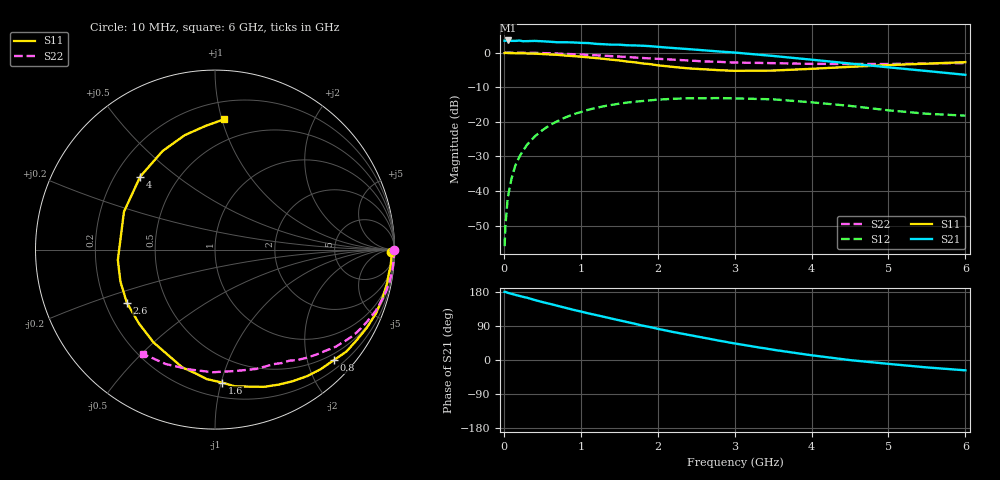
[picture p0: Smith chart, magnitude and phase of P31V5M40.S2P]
! SIEMENS Small Signal Semiconductors
! BFP181
! Si NPN RF Bipolar Junction Transistor in SOT143
! VCE = 1.5 V  IC = 0.4 mA
! Common Emitter S-Parameters:  March  1996
# GHz  S  MA  R  50
!  f  S11  S21  S12  S22
! GHz  MAG  ANG  MAG  ANG  MAG  ANG  MAG  ANG
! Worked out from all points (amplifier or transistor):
!   36 points, 10 MHz to 6 GHz, reference 50 ohm
!   highest |S21| = 3.5 dB at 50 MHz (marker M1)
!   |S21| within 3 dB of that: start of sweep to 2.69 GHz
!   unconditionally stable (mu >= 1): 3.807 GHz to end of sweep
!   at 250 MHz: K = 0.07, MSG = 15.8 dB, |S12| = -28.3 dB
!   at 1.4 GHz: K = 0.44, MSG = 8.7 dB, |S12| = -15.1 dB
!   at 6 GHz: K = 1.54, MAG = 1.6 dB, |S12| = -18.2 dB
!   S11 on the Smith chart (normalised r, x): 10 MHz: 76, -51; 800 MHz: 0.37, -2.50; 1.6 GHz: 0.31, -1.01; 2.6 GHz: 0.29, -0.26; 4 GHz: 0.30, +0.37; 6 GHz: 0.33, +1.01
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0.01  0.9821 -0.7  1.481 179.9  0.0016 87.2  0.9998 -0.2
0.02  0.9895 -1.2  1.482 179.7  0.0031 88.7  0.9928 -0.5
0.05  0.9844 -2.5  1.495 177.4  0.0079 90.7  0.9989 -1.4
0.1  0.9824 -5.5  1.475 174.7  0.0151 86.0  0.9975 -2.7
0.15  0.9773 -8.2  1.472 171.9  0.0235 84.6  0.9964 -4.0
0.2  0.9772 -10.8  1.49 169.2  0.031 81.9  0.9954 -5.4
0.3  0.9711 -16.3  1.461 164.5  0.0463 78.1  0.9931 -8.0
0.5  0.9514 -27.2  1.455 152.9  0.0755 70.4  0.9821 -13.3
0.8  0.9044 -42.9  1.408 137.8  0.1156 58.7  0.9582 -20.9
1.1  0.8514 -59.5  1.371 123.0  0.1495 47.7  0.9244 -28.2
1.3  0.8117 -70.4  1.319 114.0  0.1677 40.9  0.9012 -32.7
1.5  0.77 -81.7  1.3 104.8  0.1826 34.6  0.8744 -36.8
1.6  0.742 -86.9  1.274 100.3  0.1895 31.9  0.8646 -38.6
1.9  0.6806 -105.6  1.237 86.9  0.204 22.8  0.8225 -44.5
2.2  0.6203 -123.5  1.162 73.9  0.2149 14.9  0.7902 -49.7
2.6  0.5733 -149.0  1.078 58.7  0.2187 5.3  0.7448 -56.2
3  0.5444 -173.9  1 43.7  0.2179 -4.2  0.7172 -62.8
3.5  0.5494 157.4  0.893 27.1  0.2112 -13.6  0.7035 -70.9
4  0.5823 135.7  0.789 12.5  0.1911 -21.3  0.6859 -80.5
4.5  0.622 118.0  0.694 -0.3  0.1697 -27.1  0.6834 -91.1
5.5  0.6914 94.3  0.541 -19.6  0.1306 -26.3  0.6938 -113.2
6  0.7272 86.1  0.477 -27.3  0.1227 -21.4  0.7059 -124.5
